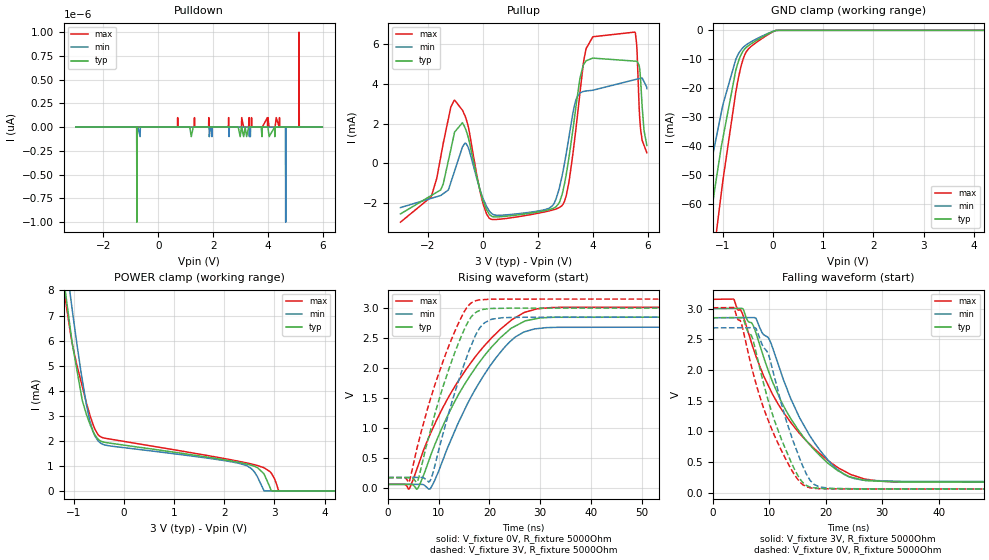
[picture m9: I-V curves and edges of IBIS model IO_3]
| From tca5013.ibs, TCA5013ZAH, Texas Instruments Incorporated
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[Model]   IO_3
Model_type   I/O
Polarity   Non-Inverting
Enable   Active-Low
Vinl = 1.2
Vinh = 1.8
Vmeas = 1.5
Vref = 3
Cref = 1pF
Rref = 5000
|   typ   min   max
C_comp   0.819p   0.538p   1.031p
|C_comp (ON state)   0.835p   0.552p   1.076p
|C_comp (OFF state)   0.819p   0.538p   1.031p
[Model spec]
|subparameter
Vinl   1.2   1.14   1.26
Vinh   1.8   1.71   1.89
[Voltage Range]   3   2.85   3.15
[Temperature Range]   27   125   -40
[Pullup Reference]   3   2.85   3.15
[Pulldown Reference]   0   0   0
[Power Clamp Reference]   3   2.85   3.15
[GND Clamp Reference]   0   0   0
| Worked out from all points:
|   slope of the pullup table from 0 to 0.45 V, typ, clamps not added: 529 ohm
|   GND clamp passes 1 mA (typ) near -0.07 V on its own axis
|   falling waveform, V_fixture 3V, R_fixture 5000Ohm: 20-80 % time 9.38ns typ, 8.07ns min, 10.9ns max; typ from 3 V to 0.174 V
|   rising waveform, V_fixture 0V, R_fixture 5000Ohm: 20-80 % time 11.1ns typ, 9.84ns min, 12.5ns max; typ from 0.062 V to 2.85 V
|   rising waveform, V_fixture 3V, R_fixture 5000Ohm: 20-80 % time 6.31ns typ, 5.88ns min, 6.86ns max; typ from 0.173 V to 3 V
|   falling waveform, V_fixture 0V, R_fixture 5000Ohm: 20-80 % time 5.67ns typ, 5.13ns min, 6.45ns max; typ from 2.85 V to 0.062 V
[Pulldown]
|   Voltage   I(typ)   I(min)   I(max)
-3V       0A         0A         0A
-786mV    0A         0A         0A
-777mV    -1pA       0A         0A
-768mV    0A         0A         0A
-660mV    0A         -100fA     0A
4.632V    0A         0A         0A
4.641V    0A         -1pA       0A
4.65V     0A         0A         0A
5.118V    0A         0A         0A
5.127V    0A         0A         1pA
5.136V    0A         0A         0A
5.973V    0A         0A         0A
[GND Clamp]
|   Voltage   I(typ)   I(min)   I(max)
-3V       -436.5mA   -240.6mA   -708.5mA
-1.47V    -93.43mA   -68.79mA   -119.6mA
-1.38V    -81.58mA   -60.02mA   -106.3mA
-1.254V   -66.24mA   -47.74mA   -88mA
-1.164V   -55.36mA   -40mA      -74.96mA
-1.029V   -40.15mA   -28.39mA   -56.2mA
-741mV    -13.86mA   -10.06mA   -21.43mA
-615mV    -7.747mA   -6.31mA    -11.13mA
-480mV    -5.182mA   -4.41mA    -6.278mA
-102mV    -1.27mA    -1.087mA   -1.504mA
141mV     0A         0A         0A
5.973V    0A         0A         0A
[Pullup]
|   Voltage   I(typ)   I(min)   I(max)
-3V       -2.533mA   -2.215mA   -2.947mA
-1.875V   -1.607mA   -1.749mA   -1.658mA
-1.029V   1.572mA    -383.4uA   3.167mA
-615mV    1.68mA     1.002mA    2.267mA
231mV     -2.54mA    -2.372mA   -2.741mA
2.877V    -1.604mA   -690.8uA   -2.123mA
3.39V     2.828mA    3.179mA    1.733mA
3.678V    4.982mA    3.616mA    5.172mA
4.011V    5.284mA    3.674mA    6.356mA
5.541V    5.134mA    4.205mA    6.59mA
5.748V    4.153mA    4.275mA    1.689mA
5.973V    905.5uA    3.753mA    534uA
[POWER Clamp]
|   Voltage   I(typ)   I(min)   I(max)
-3V       40.05mA    40.63mA    43.1mA
-1.227V   8.974mA    10.31mA    8.725mA
-1.164V   7.969mA    9.34mA     7.651mA
-1.047V   6.195mA    7.545mA    6.098mA
-826.3mV  3.607mA    4.44mA     4.168mA
-669mV    2.64mA     2.741mA    2.992mA
-426mV    1.963mA    1.868mA    2.131mA
2.283V    1.143mA    1.106mA    1.186mA
2.661V    931.7uA    571.1uA    1.015mA
2.796V    672.4uA    0A         923.2uA
3.084V    0A         0A         11.71uA
5.973V    0A         0A         0A
[Ramp]
R_load = 5000
|   typ   min   max
dV/dt_r   1.67258/1.10908e-08   1.5736/9.85439e-09   1.76966/1.24515e-08
dV/dt_f   1.69575/9.38592e-09   1.60262/8.0549e-09   1.78523/1.0948e-08
[Falling Waveform]
V_fixture = 3V
V_fixture_min = 2.85V
V_fixture_max = 3.15V
R_fixture = 5000Ohm
C_fixture = 0F
|   Time   V(typ)   V(min)   V(max)
0s        3V         2.85V      3.15V
3.795ns   3.002V     2.851V     3.145V
5.399ns   2.993V     2.852V     2.883V
7.671ns   2.6V       2.841V     2.222V
10.72ns   1.78V      2.332V     1.585V
15.09ns   1.031V     1.281V     999.7mV
20.56ns   473.5mV    520.1mV    518.2mV
24.47ns   258.1mV    252.8mV    299mV
32.33ns   180.3mV    191.4mV    179.7mV
99.9ns    173.6mV    178.7mV    174.5mV
[Rising Waveform]
V_fixture = 0V
V_fixture_min = 0V
V_fixture_max = 0V
R_fixture = 5000Ohm
C_fixture = 0F
|   Time   V(typ)   V(min)   V(max)
0s        61.74mV    62.71mV    62.77mV
4.149ns   61.48mV    62.29mV    -14.1mV
5.831ns   -8.897mV   62.12mV    354.6mV
8.27ns    513.2mV    -13.81mV   891.7mV
12.85ns   1.396V     891.8mV    1.65V
17.64ns   2.055V     1.71V      2.235V
22.67ns   2.545V     2.316V     2.683V
26.89ns   2.78V      2.603V     2.928V
35.13ns   2.846V     2.679V     3.013V
99.9ns    2.849V     2.685V     3.012V
[Rising Waveform]
V_fixture = 3V
V_fixture_min = 2.85V
V_fixture_max = 3.15V
R_fixture = 5000Ohm
C_fixture = 0F
|   Time   V(typ)   V(min)   V(max)
0s        173.5mV    178.5mV    174.5mV
4.149ns   173.2mV    178.5mV    105.8mV
5.831ns   120.1mV    178.5mV    708.9mV
8.27ns    931.6mV    119.1mV    1.463V
10.91ns   1.713V     929.7mV    2.132V
14.01ns   2.441V     1.817V     2.771V
17.18ns   2.92V      2.534V     3.119V
19.05ns   2.982V     2.756V     3.142V
22.67ns   2.996V     2.84V      3.15V
99.9ns    3V         2.85V      3.15V
[Falling Waveform]
|Gnd
V_fixture = 0V
V_fixture_min = 0V
V_fixture_max = 0V
R_fixture = 5000Ohm
C_fixture = 0F
|   Time   V(typ)   V(min)   V(max)
0s        2.849V     2.686V     3.012V
3.815ns   2.852V     2.687V     3.005V
5.399ns   2.842V     2.688V     2.641V
7.671ns   2.292V     2.677V     1.778V
9.923ns   1.475V     2.239V     1.16V
12.2ns    865.3mV    1.442V     687.7mV
14.56ns   370.2mV    765.4mV    287.3mV
16.66ns   118.4mV    297.3mV    99.31mV
21.03ns   69.4mV     74.06mV    67.64mV
99.9ns    61.75mV    62.73mV    62.77mV
